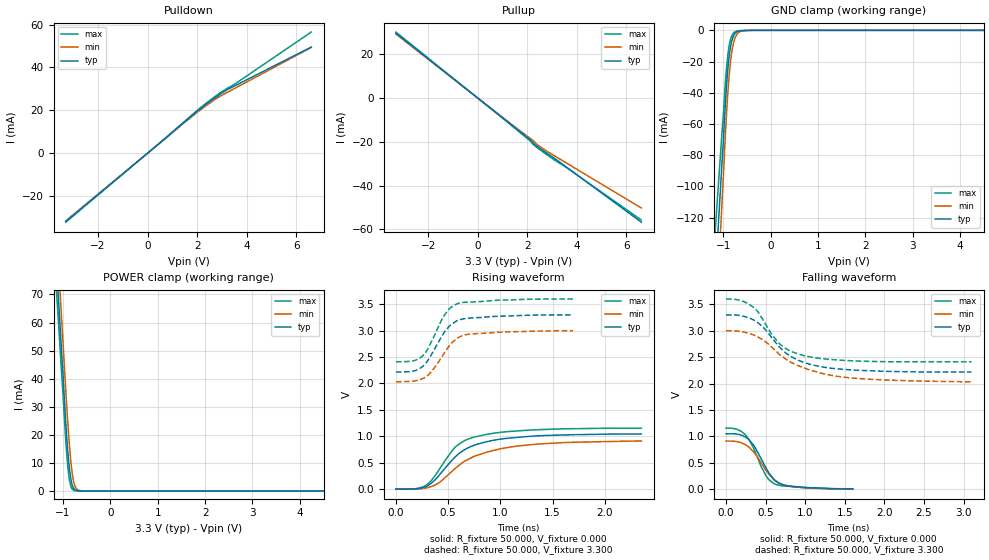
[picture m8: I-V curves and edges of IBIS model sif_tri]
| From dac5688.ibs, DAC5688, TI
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[Model]   sif_tri
Model_type 3-state
Vref=0.000E+00
Rref=1.000E+06
Cref=0.000E+00
Vmeas=1.650E+00
C_comp   5.910E-13   5.910E-13   5.910E-13
[Voltage Range]   3.300E+00   3.000E+00   3.600E+00
[POWER Clamp Reference]   3.300E+00   3.000E+00   3.600E+00
[GND Clamp Reference]   0.000E+00   0.000E+00   0.000E+00
[Pullup Reference]   3.300E+00   3.000E+00   3.600E+00
[Pulldown Reference]   0.000E+00   0.000E+00   0.000E+00
[Temperature Range]   25   85   -40
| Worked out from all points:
|   slope of the pulldown table from 0 to 0.495 V, typ, clamps not added: 103 ohm
|   slope of the pullup table from 0 to 0.495 V, typ, clamps not added: 112 ohm
|   GND clamp passes 1 mA (typ) near -0.72 V on its own axis
|   POWER clamp passes 1 mA (typ) near -0.78 V on its own axis
|   rising waveform, R_fixture 50.000, V_fixture 0.000: 20-80 % time 363ps typ, 475ps min, 297ps max; typ from 0 V to 1.04 V
|   falling waveform, R_fixture 50.000, V_fixture 0.000: 20-80 % time 245ps typ, 267ps min, 220ps max; typ from 1.05 V to 0.007 V
|   rising waveform, R_fixture 50.000, V_fixture 3.300: 20-80 % time 206ps typ, 217ps min, 186ps max; typ from 2.22 V to 3.3 V
|   falling waveform, R_fixture 50.000, V_fixture 3.300: 20-80 % time 468ps typ, 644ps min, 369ps max; typ from 3.3 V to 2.22 V
[GND Clamp]
-3.3V     -1.26A     -1.462A    -1.058A
-1.02V    -81.57mA   -106.5mA   -62.96mA
-1V       -72.25mA   -95.48mA   -55.35mA
-940mV    -39.59mA   -58.46mA   -27.39mA
-920mV    -31mA      -48mA      -20.52mA
-880mV    -17.84mA   -30.76mA   -10.73mA
-820mV    -6.793mA   -13.92mA   -3.536mA
-780mV    -3.338mA   -7.672mA   -1.598mA
-740mV    -1.582mA   -4.057mA   -730uA
-640mV    -301.7uA   -777.5uA   -204.3uA
-460mV    -50.31uA   -64.26uA   -45.47uA
6.6V      0A         0A         0A
[Power Clamp]
-3.3V     695.5mA    720.6mA    655.6mA
-1.02V    46.83mA    58.74mA    39.48mA
-940mV    23.85mA    35.39mA    17.58mA
-900mV    14.19mA    24.68mA    8.948mA
-880mV    10.42mA    19.82mA    5.833mA
-840mV    4.91mA     11.5mA     2.007mA
-820mV    3.044mA    8.223mA    1.063mA
-780mV    983.4uA    3.643mA    269.2uA
-760mV    534.8uA    2.275mA    136.7uA
-720mV    165.5uA    838.5uA    40.84uA
-620mV    28.5uA     74.19uA    5.15uA
6.6V      0A         0A         0A
[Pullup]
-3.3V     29.65mA    29.26mA    30.17mA
800mV     -7.21mA    -7.042mA   -7.309mA
2.12V     -19.11mA   -18.46mA   -19.66mA
2.26V     -20.9mA    -19.71mA   -21.42mA
2.48V     -22.81mA   -21.96mA   -23.38mA
3.14V     -27.92mA   -26.72mA   -28.66mA
3.46V     -30.59mA   -28.9mA    -30.86mA
6.6V      -56.78mA   -50.29mA   -55.79mA
[Pulldown]
-3.3V     -31.83mA   -31.54mA   -32.18mA
1.46V     14.3mA     14.02mA    14.53mA
2.54V     24.43mA    23.62mA    24.88mA
3.26V     29.92mA    28.65mA    30.56mA
3.54V     31.55mA    30.38mA    32.42mA
6.6V      49.51mA    49.32mA    56.48mA
[Rising Waveform]
R_fixture = 50.000
V_fixture = 0.000
V_fixture_min = 0.000
V_fixture_max = 0.000
|  time   V(typ)   V(min)   V(max)
0s        0V         0V         0V
190ps     4.289mV    1.454mV    7.914mV
285ps     43.9mV     18.66mV    64.83mV
340ps     111.4mV    47.34mV    162.1mV
425ps     286.7mV    135.9mV    403.2mV
565ps     604.5mV    384.5mV    789.9mV
750ps     831.2mV    619.5mV    984.5mV
995ps     944.1mV    759.8mV    1.073V
1.285ns   999.1mV    838.8mV    1.118V
2.35ns    1.043V     910.3mV    1.154V
[Falling Waveform]
R_fixture = 50.000
V_fixture = 0.000
V_fixture_min = 0.000
V_fixture_max = 0.000
|  time   V(typ)   V(min)   V(max)
0s        1.048V     910.3mV    1.154V
175ps     1.031V     887.1mV    1.108V
290ps     936.1mV    796.4mV    940.1mV
360ps     806.5mV    682.8mV    733.9mV
445ps     572.8mV    497.6mV    424.2mV
500ps     414.8mV    365.2mV    266.4mV
610ps     181mV      168.4mV    102.8mV
695ps     96.06mV    97.79mV    66.97mV
820ps     56.15mV    53.1mV     49.8mV
1.6ns     6.653mV    0V         0V
[Rising Waveform]
R_fixture = 50.000
V_fixture = 3.300
V_fixture_min = 3.000
V_fixture_max = 3.600
|  time   V(typ)   V(min)   V(max)
0s        2.218V     2.034V     2.413V
170ps     2.237V     2.046V     2.43V
250ps     2.314V     2.087V     2.513V
300ps     2.421V     2.146V     2.636V
335ps     2.53V      2.215V     2.774V
470ps     2.991V     2.596V     3.312V
520ps     3.102V     2.737V     3.431V
585ps     3.191V     2.855V     3.511V
745ps     3.244V     2.942V     3.546V
1.695ns   3.3V       3V         3.6V
[Falling Waveform]
R_fixture = 50.000
V_fixture = 3.300
V_fixture_min = 3.000
V_fixture_max = 3.600
|  time   V(typ)   V(min)   V(max)
0s        3.3V       3V         3.6V
190ps     3.286V     2.985V     3.569V
370ps     3.186V     2.906V     3.413V
475ps     3.058V     2.817V     3.188V
575ps     2.874V     2.694V     2.934V
675ps     2.69V      2.55V      2.753V
815ps     2.516V     2.406V     2.613V
985ps     2.401V     2.296V     2.528V
1.58ns    2.258V     2.106V     2.432V
3.1ns     2.218V     2.034V     2.413V
[Ramp]
dV/dt_r   6.2470E-01/3.6246E-10   5.4256E-01/4.7377E-10   6.8962E-01/2.9559E-10
dV/dt_f   6.4939E-01/4.6635E-10   5.7979E-01/6.4223E-10   7.1207E-01/3.6728E-10
R_load = 50
